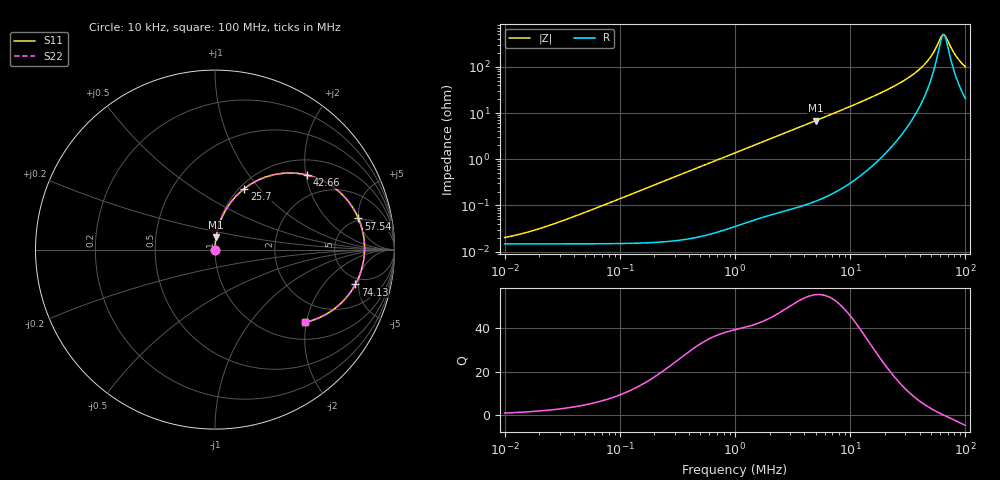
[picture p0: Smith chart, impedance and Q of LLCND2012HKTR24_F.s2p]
! LLCND2012HKTR24_F  S-PARAMETER MODEL  ( Standard Model )
! Model Generated by TAIYO YUDEN Corporation (http://www.ty-top.com)
! Version 1.0
! TAIYO YUDEN Control No. 220701
! Copyright(c) 2022 TAIYO YUDEN CO.,LTD. All Rights Reserved.
! Product Description (link to TY-COMPAS)
! https://ds.yuden.co.jp/TYCOMPAS/or/detail?pn=LLCND2012HKTR24MF&u=M
! Products Name : Inductors
! Characteristics :
!  Inductance : 0.24 [uH] , SRF(min) : - [Hz] , DC Resistance(max) : 19 [mOhm]
!  Rated Current : Saturation  7.0 [A] (dL = 30 [%]), Temp Rise  5.4 [A] (dT = 40 [degC])
!  Case Size : 2.0 x 1.2 / 0.079 x 0.047 [mm/inch] , Thickness : 0.8 / 0.031 [mm/inch]
!  (Conditions: Temperature = 25 [degC] , DC Bias Current = 0 [A])
! External Node Assignments :
!  1  o---GGG---o  2
! GND o---------o GND
! Frequency Range : 10kHz  -  100MHz  [ 402 STEP ]
# MHz S RI R 50
! Freq[MHz].  S11 Real  S11 Imag  S21 Real  S21 Imag  S12 Real  S12 Imag  S22 Real  S22 Imag
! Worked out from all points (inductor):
!   401 points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, 10 kHz to 100 MHz, reference 50 ohm
!   read as one part in series: L = 221 nH near 32.36 kHz
!   highest Q = 55.4 at 5.012 MHz (marker M1), where L = 217 nH
!   self-resonance near 64.72 MHz
!   S11 on the Smith chart (normalised r, x): 10 kHz: 1.00, +0.00; 25.7 MHz: 1.05, +0.83; 42.66 MHz: 1.38, +2.03; 57.54 MHz: 4.70, +4.94; 74.13 MHz: 4.12, -4.56; 100 MHz: 1.41, -1.95
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0.01  0.000147 0.000139  0.9999 -0.000139  0.9999 -0.000139  0.000147 0.000139
0.019055  0.000147 0.000265  0.9999 -0.000265  0.9999 -0.000265  0.000147 0.000265
0.046774  0.000148 0.000649  0.9999 -0.000649  0.9999 -0.000649  0.000148 0.000649
0.218776  0.00017 0.00304  0.9998 -0.00304  0.9998 -0.00304  0.00017 0.00304
1  0.00054 0.0138  0.9995 -0.0138  0.9995 -0.0138  0.00054 0.0138
4.677351  0.00517 0.0632  0.9948 -0.0632  0.9948 -0.0632  0.00517 0.0632
5.011872  0.00585 0.0678  0.9942 -0.0678  0.9942 -0.0678  0.00585 0.0678
11.22019  0.0274 0.1518  0.9726 -0.1518  0.9726 -0.1518  0.0274 0.1518
16.2181  0.0589 0.2193  0.9411 -0.2193  0.9411 -0.2193  0.0589 0.2193
21.87762  0.1132 0.2934  0.8868 -0.2934  0.8868 -0.2934  0.1132 0.2934
25.70396  0.1631 0.3395  0.8369 -0.3395  0.8369 -0.3395  0.1631 0.3395
33.11311  0.293 0.4078  0.707 -0.4078  0.707 -0.4078  0.293 0.4078
42.65795  0.5126 0.4156  0.4874 -0.4156  0.4874 -0.4156  0.5126 0.4156
50.11872  0.6838 0.3295  0.3162 -0.3295  0.3162 -0.3295  0.6838 0.3295
53.70318  0.7491 0.2606  0.2509 -0.2606  0.2509 -0.2606  0.7491 0.2606
57.54399  0.7995 0.1735  0.2005 -0.1735  0.2005 -0.1735  0.7995 0.1735
61.6595  0.8283 0.0735  0.1717 -0.0735  0.1717 -0.0735  0.8283 0.0735
64.56542  0.8334 0.00336  0.1666 -0.00336  0.1666 -0.00336  0.8334 0.00336
67.6083  0.8269 -0.0663  0.1731 0.0663  0.1731 0.0663  0.8269 -0.0663
74.13102  0.7821 -0.1941  0.2179 0.1941  0.2179 0.1941  0.7821 -0.1941
85.1138  0.6613 -0.3327  0.3387 0.3327  0.3387 0.3327  0.6613 -0.3327
100  0.4989 -0.406  0.5011 0.406  0.5011 0.406  0.4989 -0.406
